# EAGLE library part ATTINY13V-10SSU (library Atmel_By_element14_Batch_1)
8-bit Microcontroller with In-System Programmable Flash
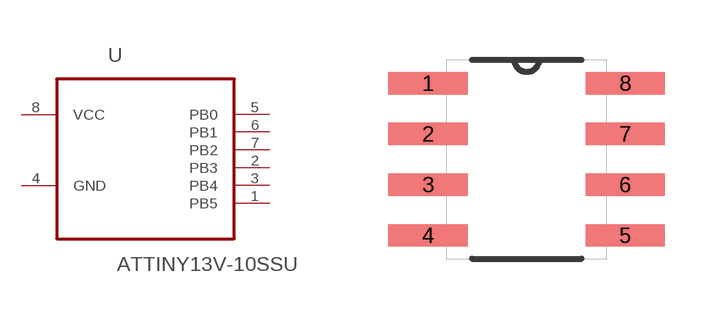
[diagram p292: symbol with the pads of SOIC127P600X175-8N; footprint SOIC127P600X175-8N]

Designator prefix U

## ATTINY13V-10SSU (MPN: ATTINY13V-10SSU; OC_FARNELL: 1455135; OC_NEWARK: 58M3773; PACKAGE: SOIC-8; SUPPLIER: Atmel)  [SOIC127P600X175-8N]
1  PB5
2  PB3
3  PB4
4  GND  pas
5  PB0
6  PB1
7  PB2
8  VCC  pwr

## Footprint SOIC127P600X175-8N (pad centres in mm)
smd 1.981 x 0.559: 1 -2.464,1.905; 2 -2.464,0.635; 3 -2.464,-0.635; 4 -2.464,-1.905; 5 2.464,-1.905; 6 2.464,-0.635; 7 2.464,0.635; 8 2.464,1.905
